|   stm32f745_746_756_tfbga216 IBIS Model
[IBIS ver]   4.2
[File name]  stm32f745_746_756_tfbga216.ibs
[File Rev]   1.0
[Date]   24-06-2015
[Source] Data Created at STMicroelectronics
[Notes]   File originated from ELDO simulations.
[Disclaimer]  This information is for modeling purpose only and is
   not guaranted. The information is subject to change without
   notice.
[Copyright] Copyright 2015 STMicroelectronics Inc.
[Component] stm32f745_746_756_tfbga216
[Manufacturer] STMicroelectronics
[Package]
| variable   typ   min   max
R_pkg   0.0   NA   NA
L_pkg   0.0H   NA   NA
C_pkg   0.0F   NA   NA
[Pin]   signal_name   model_name   R_pin   L_pin   C_pin
A1 PE4 io8p_arsudq_ft
A10 PB3 io8p_arsudq_ft
A11 PD7 io8p_arsudq_ft
A12 PC12 io8p_arsudq_ft
A13 PA15 io8p_arsudq_ft
A14 PA14 io8p_arsudq_ft
A15 PA13 io8p_arsudq_ft
A2 PE3 io8p_arsudq_ft
A3 PE2 io8p_arsudq_ft
A4 PG14 io8p_arsudq_ft
A5 PE1 io8p_arsudq_ft
A6 PE0 io8p_arsudq_ft
A7 PB8 io8p_arsudq_i2cin_ft
A8 PB5 io8p_ar3wsudq_ft
A9 PB4 io8p_arsudq_ft
B1 PE5 io8p_arsudq_ft
B10 PJ12 io8p_arsudq_ft
B11 PD6 io8p_arsudq_ft
B12 PD0 io8p_arsudq_ft
B13 PC11 io8p_arsudq_ft
B14 PC10 io8p_arsudq_ft
B15 PA12 io8usb_lsfs_otg_ft
B2 PE6 io8p_arsudq_ft
B3 PG13 io8p_arsudq_ft
B4 PB9 io8p_arsudq_i2cin_ft
B5 PB7 io8p_arsudq_i2cin_ft
B6 PB6 io8p_arsudq_i2cin_ft
B7 PG15 io8p_arsudq_ft
B8 PG11 io8p_arsudq_ft
B9 PJ13 io8p_arsudq_ft
C1 VBAT POWER
C10 PD5 io8p_arsudq_ft
C11 PD3 io8p_arsudq_ft
C12 PD1 io8p_arsudq_ft
C13 PI3 io8p_arsudq_ft
C14 PI2 io8p_arsudq_ft
C15 PA11 io8usb_lsfs_otg_ft
C2 PI8-ANTI_TAMP2  io8p_arsudq_ft_v33
C3 PI4 io8p_arsudq_ft
C4 PK7 io8p_arsudq_ft
C5 PK6 io8p_arsudq_ft
C6 PK5 io8p_arsudq_ft
C7 PG12 io8p_arsudq_ft
C8 PG10 io8p_arsudq_ft
C9 PJ14 io8p_arsudq_ft
D1 PC13-ANTI_TAMP io8p_arwsudq_ft_v33
D10 PJ15 io8p_arsudq_ft
D11 PD4 io8p_arsudq_ft
D12 PD2 io8p_arsudq_ft
D13 PH15 io8p_arsudq_ft
D14 PI1 io8p_arsudq_ft
D15 PA10 io8usb_id_otg_ft
D2 PF0 io8p_arsudq_i2cin_ft
D3 PI5 io8p_arsudq_ft
D4 PI7 io8p_arsudq_ft
D5 PI10 io8p_arsudq_ft
D6 PI6 io8p_arsudq_ft
D7 PK4 io8p_arsudq_ft
D8 PK3 io8p_arsudq_ft
D9 PG9 io8p_arsudq_ft
E1 PC14-OSC32_IN io8p_arwsudq_ft_v33
E10 VDD POWER
E11 VCAP2 POWER
E12 PH13 io8p_arsudq_ft
E13 PH14 io8p_arsudq_ft
E14 PI0 io8p_arsudq_ft
E15 PA9 io8usb_vbus_otg_ft
E2 PF1 io8p_arsudq_i2cin_ft
E3 PI12 io8p_arsudq_ft
E4 PI9 io8p_arsudq_ft
E5 PDR_ON NC
E6 BOOT vpp_test_hv
E7 VDD POWER
E8 VDD POWER
E9 VDD POWER
F1 PC15-OSC32_OUT GND
F10 VSS GND
F11 VDD POWER
F12 PK1 io8p_arsudq_ft
F13 PK2 io8p_arsudq_ft
F14 PC9 io8p_arsudq_i2cin_ft
F15 PA8 io8p_arsudq_i2cin_ft
F2 VSS  POWER
F3 PI11 io8p_arsudq_ft_v33
F4 VDD POWER
F5 VDD POWER
F6 VSS GND
F7 VSS GND
F8 VSS GND
F9 VSS GND
G1 PH0-OSC_IN io8p_arsudq_ft
G10 VSS GND
G11 VDDUSB POWER
G12 PJ11 io8p_arsudq_ft
G13 PK0 io8p_arsudq_ft
G14 PC8 io8p_arsudq_ft
G15 PC7 io8p_arsudq_ft
G2 PF2 io8p_arsudq_ft
G3 PI13 io8p_arsudq_ft
G4 PI15 io8p_arsudq_ft
G5 VDD POWER
G6 VSS  GND
H1 PH1-OSC_OUT io8p_arsudq_ft
H10 VSS GND
H11 VDD POWER
H12 PJ8 io8p_arsudq_ft
H13 PJ10 io8p_arsudq_ft
H14 PG8 io8p_arsudq_ft
H15 PC6 io8p_arsudq_ft
H2 PF3 io8p_arwsudq_ft
H3 PI14 io8p_arsudq_ft
H4 PH4 io8p_arsudq_i2cin_ft
H5 VDD POWER
H6 VSS GND
J1 NRST ioreset_ft_v33
J10 VSS GND
J11 VDD POWER
J12 PJ7 io8p_arsudq_ft
J13 PJ9 io8p_arsudq_ft
J14 PG7 io8p_arsudq_ft
J15 PG6 io8p_arsudq_ft
J2 PF4 io8p_arwsudq_ft
J3 PH5 io8p_arsudq_i2cin_ft
J4 PH3 io8p_arsudq_ft
J5 VDD POWER
J6 VSS GND
K1 PF7 io8p_arwsudq_ft
K10 VSS GND
K11 VDD POWER
K12 PJ6 io8p_arsudq_ft
K13 PD15 io8p_arsudq_ft
K14 PB13 io8usb_vbus_otg_ft
K15 PD10 io8p_arsudq_ft
K2 PF6 io8p_arwsudq_ft
K3 PF5 io8p_arwsudq_ft
K4 PH2 io8p_arsudq_ft
K5 VDD POWER
K6 VSS GND
K7 VSS GND
K8 VSS POWER
K9 VSS GND
L1 PF10 io8p_arwsudq_ft
L10 VDD POWER
L11 VCAP1 POWER
L12 PD14 io8p_arsudq_ft
L13 PB12 io8usb_id_otg_ft
L14 PD9 io8p_arsudq_ft
L15 PD8 io8p_arsudq_ft
L2 PF9 io8p_arwsudq_ft
L3 PF8 io8p_arwsudq_ft
L4 PC3 io8p_ar3wsudq_ft
L5 BYPASS_REG NC
L6 VSS GND
L7 VDD POWER
L8 VDD POWER
L9 VDD POWER
M1 VSSA GND
M10 PD12 io8p_arsudq_i2cin_ft
M11 PD13 io8p_arsudq_i2cin_ft
M12 PG3 io8p_arsudq_ft
M13 PG2 io8p_arsudq_ft
M14 PJ5 io8p_arsudq_ft
M15 PH12 io8p_arsudq_i2cin_ft
M2 PC0 io8p_ar3wsudq_ft
M3 PC1 io8p_ar3wsudq_ft_v33
M4 PC2 io8p_ar3wsudq_ft
M5 PB2 io8p_ar3wsudq_ft
M6 PF12 io8p_arsudq_ft
M7 PG1 io8p_arsudq_ft
M8 PF15 io8p_arsudq_i2cin_ft
M9 PJ4 io8p_arsudq_ft
N1 VREF- GND
N10 PD11 io8p_arsudq_ft
N11 PG5 io8p_arsudq_ft
N12 PG4 io8p_arsudq_ft
N13 PH7 io8p_arsudq_i2cin_ft
N14 PH9 io8p_arsudq_ft
N15 PH11 io8p_arsudq_i2cin_ft
N2 PA1 io8p_ar3wsudq_ft
N3 PA0-WKUP io8p_ar3wsudq_ft_v33
N4 PA4 io8p_ar3wsudq_ft
N5 PC4 io8p_ar3wsudq_ft
N6 PF13 io8p_arsudq_ft
N7 PG0 io8p_arsudq_ft
N8 PJ3 io8p_arsudq_ft
N9 PE8 io8p_arsudq_ft
P1 VREF+ POWER
P10 PE11 io8p_arsudq_ft
P11 PE14 io8p_arsudq_ft
P12 PB10 io8p_arsudq_i2cin_ft
P13 PH6 io8p_arsudq_ft
P14 PH8 io8p_arsudq_i2cin_ft
P15 PH10 io8p_arsudq_ft
P2 PA2 io8p_ar3wsudq_ft_v33
P3 PA6 io8p_ar3wsudq_ft
P4 PA5 io8p_ar3wsudq_ft
P5 PC5 io8p_ar3wsudq_ft
P6 PF14 io8p_arsudq_i2cin_ft
P7 PJ2 io8p_arsudq_ft
P8 PF11 io8p_arsudq_ft
P9 PE9 io8p_arsudq_ft
R1 VDDA POWER
R10 PE12 io8p_arsudq_ft
R11 PE15 io8p_ar3wsudq_ft
R12 PE13 io8p_arsudq_ft
R13 PB11 io8p_arsudq_i2cin_ft
R14 PB14 io8usb_lsfs_otg_ft
R15 PB15 io8usb_lsfs_otg_ft
R2 PA3 io8p_ar3wsudq_ft
R3 PA7 io8p_ar3wsudq_ft
R4 PB1 io8p_ar3wsudq_ft
R5 PB0 io8p_ar3wsudq_ft
R6 PJ0 io8p_arsudq_ft
R7 PJ1 io8p_arsudq_ft
R8 PE7 io8p_arsudq_ft
R9 PE10 io8p_arsudq_ft
[Diff Pin]   inv_pin   vdiff   tdelay_typ  tdelay_min  tdelay_max
R14   R15   200mV   NA   NA   NA
C15   B15   200mV   NA   NA   NA
[Model Selector] io8p_ar3wsudq_ft
io8p00_ar3wsudq_ft_pd_lv  "SPEED00 1P8V, PD=40kOhm"
io8p00_ar3wsudq_ft_pu_lv  "SPEED00 1P8V, PU=40kOhm"
io8p00_ar3wsudq_ft_lv  "SPEED00 1P8V"
io8p01_ar3wsudq_ft_pd_lv  "SPEED01 1P8V, PD=40kOhm"
io8p01_ar3wsudq_ft_pu_lv  "SPEED01 1P8V, PU=40kOhm"
io8p01_ar3wsudq_ft_lv  "SPEED01 1P8V"
io8p10_ar3wsudq_ft_pd_lv  "SPEED10 1P8V, PD=40kOhm"
io8p10_ar3wsudq_ft_pu_lv  "SPEED10 1P8V, PU=40kOhm"
io8p10_ar3wsudq_ft_lv  "SPEED10 1P8V"
io8p11_ar3wsudq_ft_pd_lv  "SPEED11 1P8V, PD=40kOhm"
io8p11_ar3wsudq_ft_pu_lv  "SPEED11 1P8V, PU=40kOhm"
io8p11_ar3wsudq_ft_lv  "SPEED11 1P8V"
io8p00_ar3wsudq_ft_pd  "SPEED00, PD=40kOhm"
io8p00_ar3wsudq_ft_pu  "SPEED00, PU=40kOhm"
io8p00_ar3wsudq_ft  "SPEED00"
io8p01_ar3wsudq_ft_pd  "SPEED01, PD=40kOhm"
io8p01_ar3wsudq_ft_pu  "SPEED01, PU=40kOhm"
io8p01_ar3wsudq_ft  "SPEED01"
io8p10_ar3wsudq_ft_pd  "SPEED10, PD=40kOhm"
io8p10_ar3wsudq_ft_pu  "SPEED10, PU=40kOhm"
io8p10_ar3wsudq_ft  "SPEED10"
io8p11_ar3wsudq_ft_pd  "SPEED11, PD=40kOhm"
io8p11_ar3wsudq_ft_pu  "SPEED11, PU=40kOhm"
io8p11_ar3wsudq_ft  "SPEED11"
[Model Selector] io8p_ar3wsudq_ft_v33
io8p00_ar3wsudq_ft_v33_pd_lv  "SPEED00 1P8V, PD=40kOhm"
io8p00_ar3wsudq_ft_v33_pu_lv  "SPEED00 1P8V, PU=40kOhm"
io8p00_ar3wsudq_ft_v33_lv  "SPEED00 1P8V"
io8p01_ar3wsudq_ft_v33_pd_lv  "SPEED01 1P8V, PD=40kOhm"
io8p01_ar3wsudq_ft_v33_pu_lv  "SPEED01 1P8V, PU=40kOhm"
io8p01_ar3wsudq_ft_v33_lv  "SPEED01 1P8V"
io8p10_ar3wsudq_ft_v33_pd_lv  "SPEED10 1P8V, PD=40kOhm"
io8p10_ar3wsudq_ft_v33_pu_lv  "SPEED10 1P8V, PU=40kOhm"
io8p10_ar3wsudq_ft_v33_lv  "SPEED10 1P8V"
io8p11_ar3wsudq_ft_v33_pd_lv  "SPEED11 1P8V, PD=40kOhm"
io8p11_ar3wsudq_ft_v33_pu_lv  "SPEED11 1P8V, PU=40kOhm"
io8p11_ar3wsudq_ft_v33_lv  "SPEED11 1P8V"
io8p00_ar3wsudq_ft_v33_pd  "SPEED00, PD=40kOhm"
io8p00_ar3wsudq_ft_v33_pu  "SPEED00, PU=40kOhm"
io8p00_ar3wsudq_ft_v33  "SPEED00"
io8p01_ar3wsudq_ft_v33_pd  "SPEED01, PD=40kOhm"
io8p01_ar3wsudq_ft_v33_pu  "SPEED01, PU=40kOhm"
io8p01_ar3wsudq_ft_v33  "SPEED01"
io8p10_ar3wsudq_ft_v33_pd  "SPEED10, PD=40kOhm"
io8p10_ar3wsudq_ft_v33_pu  "SPEED10, PU=40kOhm"
io8p10_ar3wsudq_ft_v33  "SPEED10"
io8p11_ar3wsudq_ft_v33_pd  "SPEED11, PD=40kOhm"
io8p11_ar3wsudq_ft_v33_pu  "SPEED11, PU=40kOhm"
io8p11_ar3wsudq_ft_v33  "SPEED11"
[Model Selector] io8p_arsudq_ft
io8p00_arsudq_ft_pd_lv  "SPEED00 1P8V, PD=40kOhm"
io8p00_arsudq_ft_pu_lv  "SPEED00 1P8V, PU=40kOhm"
io8p00_arsudq_ft_lv  "SPEED00 1P8V"
io8p01_arsudq_ft_pd_lv  "SPEED01 1P8V, PD=40kOhm"
io8p01_arsudq_ft_pu_lv  "SPEED01 1P8V, PU=40kOhm"
io8p01_arsudq_ft_lv  "SPEED01 1P8V"
io8p10_arsudq_ft_pd_lv  "SPEED10 1P8V, PD=40kOhm"
io8p10_arsudq_ft_pu_lv  "SPEED10 1P8V, PU=40kOhm"
io8p10_arsudq_ft_lv  "SPEED10 1P8V"
io8p11_arsudq_ft_pd_lv  "SPEED11 1P8V, PD=40kOhm"
io8p11_arsudq_ft_pu_lv  "SPEED11 1P8V, PU=40kOhm"
io8p11_arsudq_ft_lv  "SPEED11 1P8V"
io8p00_arsudq_ft_pd  "SPEED00, PD=40kOhm"
io8p00_arsudq_ft_pu  "SPEED00, PU=40kOhm"
io8p00_arsudq_ft  "SPEED00"
io8p01_arsudq_ft_pd  "SPEED01, PD=40kOhm"
io8p01_arsudq_ft_pu  "SPEED01, PU=40kOhm"
io8p01_arsudq_ft  "SPEED01"
io8p10_arsudq_ft_pd  "SPEED10, PD=40kOhm"
io8p10_arsudq_ft_pu  "SPEED10, PU=40kOhm"
io8p10_arsudq_ft  "SPEED10"
io8p11_arsudq_ft_pd  "SPEED11, PD=40kOhm"
io8p11_arsudq_ft_pu  "SPEED11, PU=40kOhm"
io8p11_arsudq_ft  "SPEED11"
[Model Selector] io8p_arsudq_i2cin_ft
io8p00_arsudq_i2cin_ft_pd_lv  "SPEED00 1P8V, PD=40kOhm"
io8p00_arsudq_i2cin_ft_pu_lv  "SPEED00 1P8V, PU=40kOhm"
io8p00_arsudq_i2cin_ft_lv  "SPEED00 1P8V"
io8p01_arsudq_i2cin_ft_pd_lv  "SPEED01 1P8V, PD=40kOhm"
io8p01_arsudq_i2cin_ft_pu_lv  "SPEED01 1P8V, PU=40kOhm"
io8p01_arsudq_i2cin_ft_lv  "SPEED01 1P8V"
io8p10_arsudq_i2cin_ft_pd_lv  "SPEED10 1P8V, PD=40kOhm"
io8p10_arsudq_i2cin_ft_pu_lv  "SPEED10 1P8V, PU=40kOhm"
io8p10_arsudq_i2cin_ft_lv  "SPEED10 1P8V"
io8p11_arsudq_i2cin_ft_pd_lv  "SPEED11 1P8V, PD=40kOhm"
io8p11_arsudq_i2cin_ft_pu_lv  "SPEED11 1P8V, PU=40kOhm"
io8p11_arsudq_i2cin_ft_lv  "SPEED11 1P8V"
io8p00_arsudq_i2cin_ft_pd  "SPEED00, PD=40kOhm"
io8p00_arsudq_i2cin_ft_pu  "SPEED00, PU=40kOhm"
io8p00_arsudq_i2cin_ft  "SPEED00"
io8p01_arsudq_i2cin_ft_pd  "SPEED01, PD=40kOhm"
io8p01_arsudq_i2cin_ft_pu  "SPEED01, PU=40kOhm"
io8p01_arsudq_i2cin_ft  "SPEED01"
io8p10_arsudq_i2cin_ft_pd  "SPEED10, PD=40kOhm"
io8p10_arsudq_i2cin_ft_pu  "SPEED10, PU=40kOhm"
io8p10_arsudq_i2cin_ft  "SPEED10"
io8p11_arsudq_i2cin_ft_pd  "SPEED11, PD=40kOhm"
io8p11_arsudq_i2cin_ft_pu  "SPEED11, PU=40kOhm"
io8p11_arsudq_i2cin_ft  "SPEED11"
[Model Selector] io8p_arwsudq_ft_v33
io8p00_arwsudq_ft_v33_pd_lv  "SPEED00 1P8V, PD=40kOhm"
io8p00_arwsudq_ft_v33_pu_lv  "SPEED00 1P8V, PU=40kOhm"
io8p00_arwsudq_ft_v33_lv  "SPEED00 1P8V"
io8p01_arwsudq_ft_v33_pd_lv  "SPEED01 1P8V, PD=40kOhm"
io8p01_arwsudq_ft_v33_pu_lv  "SPEED01 1P8V, PU=40kOhm"
io8p01_arwsudq_ft_v33_lv  "SPEED01 1P8V"
io8p10_arwsudq_ft_v33_pd_lv  "SPEED10 1P8V, PD=40kOhm"
io8p10_arwsudq_ft_v33_pu_lv  "SPEED10 1P8V, PU=40kOhm"
io8p10_arwsudq_ft_v33_lv  "SPEED10 1P8V"
io8p11_arwsudq_ft_v33_pd_lv  "SPEED11 1P8V, PD=40kOhm"
io8p11_arwsudq_ft_v33_pu_lv  "SPEED11 1P8V, PU=40kOhm"
io8p11_arwsudq_ft_v33_lv  "SPEED11 1P8V"
io8p00_arwsudq_ft_v33_pd  "SPEED00, PD=40kOhm"
io8p00_arwsudq_ft_v33_pu  "SPEED00, PU=40kOhm"
io8p00_arwsudq_ft_v33  "SPEED00"
io8p01_arwsudq_ft_v33_pd  "SPEED01, PD=40kOhm"
io8p01_arwsudq_ft_v33_pu  "SPEED01, PU=40kOhm"
io8p01_arwsudq_ft_v33  "SPEED01"
io8p10_arwsudq_ft_v33_pd  "SPEED10, PD=40kOhm"
io8p10_arwsudq_ft_v33_pu  "SPEED10, PU=40kOhm"
io8p10_arwsudq_ft_v33  "SPEED10"
io8p11_arwsudq_ft_v33_pd  "SPEED11, PD=40kOhm"
io8p11_arwsudq_ft_v33_pu  "SPEED11, PU=40kOhm"
io8p11_arwsudq_ft_v33  "SPEED11"
[Model Selector] io8usb_id_otg_ft
io8p00_id_otg_ft_pd_lv  "SPEED00 1P8V, PD=14kOhm"
io8p00_id_otg_ft_pu_lv  "SPEED00 1P8V, PU=14kOhm"
io8p00_id_otg_ft_lv  "SPEED00 1P8V"
io8p01_id_otg_ft_pd_lv  "SPEED01 1P8V, PD=14kOhm"
io8p01_id_otg_ft_pu_lv  "SPEED01 1P8V, PU=14kOhm"
io8p01_id_otg_ft_lv  "SPEED01 1P8V"
io8p10_id_otg_ft_pd_lv  "SPEED10 1P8V, PD=14kOhm"
io8p10_id_otg_ft_pu_lv  "SPEED10 1P8V, PU=14kOhm"
io8p10_id_otg_ft_lv  "SPEED10 1P8V"
io8p11_id_otg_ft_pd_lv  "SPEED11 1P8V, PD=14kOhm"
io8p11_id_otg_ft_pu_lv  "SPEED11 1P8V, PU=14kOhm"
io8p11_id_otg_ft_lv  "SPEED11 1P8V"
io8p00_id_otg_ft_pd  "SPEED00, PD=14kOhm"
io8p00_id_otg_ft_pu  "SPEED00, PU=14kOhm"
io8p00_id_otg_ft  "SPEED00"
io8p01_id_otg_ft_pd  "SPEED01, PD=14kOhm"
io8p01_id_otg_ft_pu  "SPEED01, PU=14kOhm"
io8p01_id_otg_ft  "SPEED01"
io8p10_id_otg_ft_pd  "SPEED10, PD=14kOhm"
io8p10_id_otg_ft_pu  "SPEED10, PU=14kOhm"
io8p10_id_otg_ft  "SPEED10"
io8p11_id_otg_ft_pd  "SPEED11, PD=14kOhm"
io8p11_id_otg_ft_pu  "SPEED11, PU=14kOhm"
io8p11_id_otg_ft  "SPEED11"
[Model Selector] io8usb_lsfs_otg_ft
io8usb_ls_otg_ft_dpdn_pd  "LS USB DP/DN IO + PD=20kOhm"
io8usb_ls_otg_ft_dpdn_pupu2  "LS USB DP/DN IO + PU/PU2=2.2kOhm"
io8usb_ls_otg_ft_dpdn_pu2  "LS USB DP/DN IO + PU2=1.2kOhm"
io8usb_ls_otg_ft_dpdn_pu  "LS USB DP/DN IO + PU=1.2kOhm"
io8usb_ls_otg_ft_dpdn  "LS USB DP/DN IO"
io8usb_fs_otg_ft_dpdn_pd  "HS USB DP/DN IO + PD=20kOhm"
io8usb_fs_otg_ft_dpdn_pupu2  "HS USB DP/DN IO + PU/PU2=2.2kOhm"
io8usb_fs_otg_ft_dpdn_pu2  "HS USB DP/DN IO + PU2=1.2kOhm"
io8usb_fs_otg_ft_dpdn_pu  "HS USB DP/DN IO + PU=1.2kOhm"
io8usb_fs_otg_ft_dpdn  "HS USB DP/DN IO"
io8p00_lsfs_otg_ft_pd_lv  "SPEED00 1P8V, PD=40kOhm"
io8p00_lsfs_otg_ft_pu_lv  "SPEED00 1P8V, PU=40kOhm"
io8p00_lsfs_otg_ft_lv  "SPEED00 1P8V"
io8p01_lsfs_otg_ft_pd_lv  "SPEED01 1P8V, PD=40kOhm"
io8p01_lsfs_otg_ft_pu_lv  "SPEED01 1P8V, PU=40kOhm"
io8p01_lsfs_otg_ft_lv  "SPEED01 1P8V"
io8p10_lsfs_otg_ft_pd_lv  "SPEED10 1P8V, PD=40kOhm"
io8p10_lsfs_otg_ft_pu_lv  "SPEED10 1P8V, PU=40kOhm"
io8p10_lsfs_otg_ft_lv  "SPEED10 1P8V"
io8p11_lsfs_otg_ft_pd_lv  "SPEED11 1P8V, PD=40kOhm"
io8p11_lsfs_otg_ft_pu_lv  "SPEED11 1P8V, PU=40kOhm"
io8p11_lsfs_otg_ft_lv  "SPEED11 1P8V"
io8p00_lsfs_otg_ft_pd  "SPEED00, PD=40kOhm"
io8p00_lsfs_otg_ft_pu  "SPEED00, PU=40kOhm"
io8p00_lsfs_otg_ft  "SPEED00"
io8p01_lsfs_otg_ft_pd  "SPEED01, PD=40kOhm"
io8p01_lsfs_otg_ft_pu  "SPEED01, PU=40kOhm"
io8p01_lsfs_otg_ft  "SPEED01"
io8p10_lsfs_otg_ft_pd  "SPEED10, PD=40kOhm"
io8p10_lsfs_otg_ft_pu  "SPEED10, PU=40kOhm"
io8p10_lsfs_otg_ft  "SPEED10"
io8p11_lsfs_otg_ft_pd  "SPEED11, PD=40kOhm"
io8p11_lsfs_otg_ft_pu  "SPEED11, PU=40kOhm"
io8p11_lsfs_otg_ft  "SPEED11"
[Model Selector] io8usb_vbus_otg_ft
io8psenb_vbus_otg_ft  "VBUS PULSE, SENSE VB"
io8psenab_vbus_otg_ft  "VBUS PULSE, SENSE VA and VB"
io8psena_vbus_otg_ft  "VBUS PULSE, SENSE VA"
io8psen_vbus_otg_ft  "VBUS PULSE"
io8p00_vbus_otg_ft_pd_lv  "SPEED00 1P8V, PD=40kOhm"
io8p00_vbus_otg_ft_pu_lv  "SPEED00 1P8V, PU=40kOhm"
io8p00_vbus_otg_ft_lv  "SPEED00 1P8V"
io8p01_vbus_otg_ft_pd_lv  "SPEED01 1P8V, PD=40kOhm"
io8p01_vbus_otg_ft_pu_lv  "SPEED01 1P8V, PU=40kOhm"
io8p01_vbus_otg_ft_lv  "SPEED01 1P8V"
io8p10_vbus_otg_ft_pd_lv  "SPEED10 1P8V, PD=40kOhm"
io8p10_vbus_otg_ft_pu_lv  "SPEED10 1P8V, PU=40kOhm"
io8p10_vbus_otg_ft_lv  "SPEED10 1P8V"
io8p11_vbus_otg_ft_pd_lv  "SPEED11 1P8V, PD=40kOhm"
io8p11_vbus_otg_ft_pu_lv  "SPEED11 1P8V, PU=40kOhm"
io8p11_vbus_otg_ft_lv  "SPEED11 1P8V"
io8p00_vbus_otg_ft_pd  "SPEED00, PD=40kOhm"
io8p00_vbus_otg_ft_pu  "SPEED00, PU=40kOhm"
io8p00_vbus_otg_ft  "SPEED00"
io8p01_vbus_otg_ft_pd  "SPEED01, PD=40kOhm"
io8p01_vbus_otg_ft_pu  "SPEED01, PU=40kOhm"
io8p01_vbus_otg_ft  "SPEED01"
io8p10_vbus_otg_ft_pd  "SPEED10, PD=40kOhm"
io8p10_vbus_otg_ft_pu  "SPEED10, PU=40kOhm"
io8p10_vbus_otg_ft  "SPEED10"
io8p11_vbus_otg_ft_pd  "SPEED11, PD=40kOhm"
io8p11_vbus_otg_ft_pu  "SPEED11, PU=40kOhm"
io8p11_vbus_otg_ft  "SPEED11"
[Model Selector] ioreset_ft_v33
ioreset_ft_v33_pu_lv  "ioreset 1P8V + PU=40kOhm"
ioreset_ft_v33_nopu_lv  "ioreset 1P8V"
ioreset_ft_v33_pu  "ioreset + PU=40kOhm"
ioreset_ft_v33_nopu  "ioreset"
[Model Selector] vpp_test_hv
vpp_test_hv_2p4  "Input Buffer 1P8V"
vpp_test_hv_3p3  "Input Buffer"
[Model Selector] io8p_arwsudq_ft
io8p00_arwsudq_ft_pd_lv  "SPEED00 1P8V, PD=40kOhm"
io8p00_arwsudq_ft_pu_lv  "SPEED00 1P8V, PU=40kOhm"
io8p00_arwsudq_ft_lv  "SPEED00 1P8V"
io8p01_arwsudq_ft_pd_lv  "SPEED01 1P8V, PD=40kOhm"
io8p01_arwsudq_ft_pu_lv  "SPEED01 1P8V, PU=40kOhm"
io8p01_arwsudq_ft_lv  "SPEED01 1P8V"
io8p10_arwsudq_ft_pd_lv  "SPEED10 1P8V, PD=40kOhm"
io8p10_arwsudq_ft_pu_lv  "SPEED10 1P8V, PU=40kOhm"
io8p10_arwsudq_ft_lv  "SPEED10 1P8V"
io8p11_arwsudq_ft_pd_lv  "SPEED11 1P8V, PD=40kOhm"
io8p11_arwsudq_ft_pu_lv  "SPEED11 1P8V, PU=40kOhm"
io8p11_arwsudq_ft_lv  "SPEED11 1P8V"
io8p00_arwsudq_ft_pd  "SPEED00, PD=40kOhm"
io8p00_arwsudq_ft_pu  "SPEED00, PU=40kOhm"
io8p00_arwsudq_ft  "SPEED00"
io8p01_arwsudq_ft_pd  "SPEED01, PD=40kOhm"
io8p01_arwsudq_ft_pu  "SPEED01, PU=40kOhm"
io8p01_arwsudq_ft  "SPEED01"
io8p10_arwsudq_ft_pd  "SPEED10, PD=40kOhm"
io8p10_arwsudq_ft_pu  "SPEED10, PU=40kOhm"
io8p10_arwsudq_ft  "SPEED10"
io8p11_arwsudq_ft_pd  "SPEED11, PD=40kOhm"
io8p11_arwsudq_ft_pu  "SPEED11, PU=40kOhm"
io8p11_arwsudq_ft  "SPEED11"
[Model Selector] io8p_arsudq_ft_v33
io8p00_arsudq_ft_v33_pd_lv  "SPEED00 1P8V, PD=40kOhm"
io8p00_arsudq_ft_v33_pu_lv  "SPEED00 1P8V, PU=40kOhm"
io8p00_arsudq_ft_v33_lv  "SPEED00 1P8V"
io8p01_arsudq_ft_v33_pd_lv  "SPEED01 1P8V, PD=40kOhm"
io8p01_arsudq_ft_v33_pu_lv  "SPEED01 1P8V, PU=40kOhm"
io8p01_arsudq_ft_v33_lv  "SPEED01 1P8V"
io8p10_arsudq_ft_v33_pd_lv  "SPEED10 1P8V, PD=40kOhm"
io8p10_arsudq_ft_v33_pu_lv  "SPEED10 1P8V, PU=40kOhm"
io8p10_arsudq_ft_v33_lv  "SPEED10 1P8V"
io8p11_arsudq_ft_v33_pd_lv  "SPEED11 1P8V, PD=40kOhm"
io8p11_arsudq_ft_v33_pu_lv  "SPEED11 1P8V, PU=40kOhm"
io8p11_arsudq_ft_v33_lv  "SPEED11 1P8V"
io8p00_arsudq_ft_v33_pd  "SPEED00, PD=40kOhm"
io8p00_arsudq_ft_v33_pu  "SPEED00, PU=40kOhm"
io8p00_arsudq_ft_v33  "SPEED00"
io8p01_arsudq_ft_v33_pd  "SPEED01, PD=40kOhm"
io8p01_arsudq_ft_v33_pu  "SPEED01, PU=40kOhm"
io8p01_arsudq_ft_v33  "SPEED01"
io8p10_arsudq_ft_v33_pd  "SPEED10, PD=40kOhm"
io8p10_arsudq_ft_v33_pu  "SPEED10, PU=40kOhm"
io8p10_arsudq_ft_v33  "SPEED10"
io8p11_arsudq_ft_v33_pd  "SPEED11, PD=40kOhm"
io8p11_arsudq_ft_v33_pu  "SPEED11, PU=40kOhm"
io8p11_arsudq_ft_v33  "SPEED11"
| Models and submodels in the file (260): io8p00_ar3wsudq_ft_pd_lv (I/O), io8p00_ar3wsudq_ft_pu_lv (I/O), io8p00_ar3wsudq_ft_lv (I/O), io8p01_ar3wsudq_ft_pd_lv (I/O), io8p01_ar3wsudq_ft_pu_lv (I/O), io8p01_ar3wsudq_ft_lv (I/O), io8p10_ar3wsudq_ft_pd_lv (I/O), io8p10_ar3wsudq_ft_pu_lv (I/O), io8p10_ar3wsudq_ft_lv (I/O), io8p11_ar3wsudq_ft_pd_lv (I/O), io8p11_ar3wsudq_ft_pu_lv (I/O), io8p11_ar3wsudq_ft_lv (I/O), io8p00_ar3wsudq_ft_pd (I/O), io8p00_ar3wsudq_ft_pu (I/O), io8p00_ar3wsudq_ft (I/O), io8p01_ar3wsudq_ft_pd (I/O), io8p01_ar3wsudq_ft_pu (I/O), io8p01_ar3wsudq_ft (I/O), io8p10_ar3wsudq_ft_pd (I/O), io8p10_ar3wsudq_ft_pu (I/O), io8p10_ar3wsudq_ft (I/O), io8p11_ar3wsudq_ft_pd (I/O), io8p11_ar3wsudq_ft_pu (I/O), io8p11_ar3wsudq_ft (I/O), io8p00_ar3wsudq_ft_v33_pd_lv (I/O), io8p00_ar3wsudq_ft_v33_pu_lv (I/O), io8p00_ar3wsudq_ft_v33_lv (I/O), io8p01_ar3wsudq_ft_v33_pd_lv (I/O), io8p01_ar3wsudq_ft_v33_pu_lv (I/O), io8p01_ar3wsudq_ft_v33_lv (I/O), io8p10_ar3wsudq_ft_v33_pd_lv (I/O), io8p10_ar3wsudq_ft_v33_pu_lv (I/O), io8p10_ar3wsudq_ft_v33_lv (I/O), io8p11_ar3wsudq_ft_v33_pd_lv (I/O), io8p11_ar3wsudq_ft_v33_pu_lv (I/O), io8p11_ar3wsudq_ft_v33_lv (I/O), io8p00_ar3wsudq_ft_v33_pd (I/O), io8p00_ar3wsudq_ft_v33_pu (I/O), io8p00_ar3wsudq_ft_v33 (I/O), io8p01_ar3wsudq_ft_v33_pd (I/O), io8p01_ar3wsudq_ft_v33_pu (I/O), io8p01_ar3wsudq_ft_v33 (I/O), io8p10_ar3wsudq_ft_v33_pd (I/O), io8p10_ar3wsudq_ft_v33_pu (I/O), io8p10_ar3wsudq_ft_v33 (I/O), io8p11_ar3wsudq_ft_v33_pd (I/O), io8p11_ar3wsudq_ft_v33_pu (I/O), io8p11_ar3wsudq_ft_v33 (I/O), io8p00_arsudq_ft_pd_lv (I/O), io8p00_arsudq_ft_pu_lv (I/O), io8p00_arsudq_ft_lv (I/O), io8p01_arsudq_ft_pd_lv (I/O), io8p01_arsudq_ft_pu_lv (I/O), io8p01_arsudq_ft_lv (I/O), io8p10_arsudq_ft_pd_lv (I/O), io8p10_arsudq_ft_pu_lv (I/O), io8p10_arsudq_ft_lv (I/O), io8p11_arsudq_ft_pd_lv (I/O), io8p11_arsudq_ft_pu_lv (I/O), io8p11_arsudq_ft_lv (I/O), io8p00_arsudq_ft_pd (I/O), io8p00_arsudq_ft_pu (I/O), io8p00_arsudq_ft (I/O), io8p01_arsudq_ft_pd (I/O), io8p01_arsudq_ft_pu (I/O), io8p01_arsudq_ft (I/O), io8p10_arsudq_ft_pd (I/O), io8p10_arsudq_ft_pu (I/O), io8p10_arsudq_ft (I/O), io8p11_arsudq_ft_pd (I/O), io8p11_arsudq_ft_pu (I/O), io8p11_arsudq_ft (I/O), io8p00_arsudq_i2cin_ft_pd_lv (I/O), io8p00_arsudq_i2cin_ft_pu_lv (I/O), io8p00_arsudq_i2cin_ft_lv (I/O), io8p01_arsudq_i2cin_ft_pd_lv (I/O), io8p01_arsudq_i2cin_ft_pu_lv (I/O), io8p01_arsudq_i2cin_ft_lv (I/O), io8p10_arsudq_i2cin_ft_pd_lv (I/O), io8p10_arsudq_i2cin_ft_pu_lv (I/O)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
